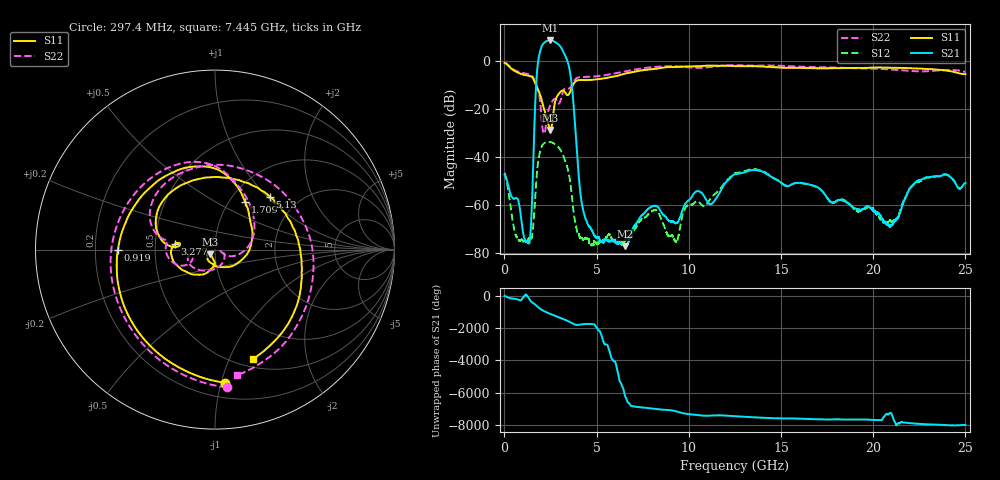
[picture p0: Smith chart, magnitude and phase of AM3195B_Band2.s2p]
!Agilent Technologies,E8364B,MY43040894,A.07.50.67
!Agilent E8364B: A.07.50.67
!Date: Wednesday, July 07, 2021 13:16:47
!Correction: S11(Full 2 Port(1,2))
!S21(Full 2 Port(1,2))
!S12(Full 2 Port(1,2))
!S22(Full 2 Port(1,2))
!S2P File: Measurements: S11, S21, S12, S22:
# Hz S  dB  R 50
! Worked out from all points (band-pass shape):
!   8001 points, 10 MHz to 25 GHz, reference 50 ohm
!   highest |S21| = 8.66 dB at 2.475 GHz (marker M1); lowest = -77.1 dB at 6.539 GHz (marker M2)
!   |S21| within 3 dB of the highest: 1.994 GHz to 3.073 GHz (1.079 GHz wide, 42.6 % of centre)
!   lowest |S11| = -28.7 dB at 2.478 GHz (marker M3), VSWR 1.08, Z = 47.4 - j2.49 ohm
!   |S11| at or under -10 dB: 1.706 GHz to 3.708 GHz (2.002 GHz wide, 73.9 % of centre)
!   |S22| runs from -30.2 to -0.5 dB; largest |S21 - S12| = 2.7
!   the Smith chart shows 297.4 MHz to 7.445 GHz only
!   S11 on the Smith chart (normalised r, x): 297.4 MHz: 0.31, -1.03; 919 MHz: 0.30, -0.00; 1.709 GHz: 1.18, +0.70; 3.277 GHz: 0.63, +0.04; 5.13 GHz: 1.44, +1.03; 7.445 GHz: 0.59, -1.23
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1e7  -0.75 -14.5  -47.39 -12.2  -46.58 -18.6  -0.51 -15.3
2.97385e8  -2.57 -85.6  -54.63 -152.2  -58.78 -157.9  -2.27 -85.2
9.190112e8  -5.33 -179.7  -66.32 99.8  -74.21 -69.9  -4.76 -179.7
1.371955e9  -6.16 121.7  -75.03 118.3  -73.86 37.3  -5.53 123.7
1.70932e9  -10.06 57.5  -11.28 123.5  -52.31 -50.5  -9.42 58.7
1.95922e9  -14.53 -3.1  4.85 -112.1  -36.96 77.6  -18.66 -16.9
2.090418e9  -18.17 -51.4  7.13 158.1  -34.70 -10.9  -29.03 -19.4
2.230986e9  -22.07 -103.9  8.15 77.2  -33.85 -90.3  -27.95 -14.8
2.474639e9  -28.66 -135.5  8.66 -42.9  -33.70 150.7  -18.55 -102.8
2.477762e9  -28.66 -134.7  8.66 -44.4  -33.70 149.3  -18.50 -103.6
2.768271e9  -16.27 -115.6  7.91 -174.7  -34.77 20.7  -15.85 -160.3
2.980686e9  -13.26 -149.6  6.62 91.0  -36.29 -71.4  -17.50 -158.4
3.277442e9  -12.89 172.3  2.64 -45.9  -41.07 155.7  -11.41 -173.7
4.177082e9  -7.86 114.8  -58.42 20.0  -73.78 130.5  -6.62 113.9
5.129826e9  -7.45 44.1  -73.47 -15.0  -75.69 -74.1  -6.15 42.6
6.538638e9  -5.20 -33.5  -77.14 -74.2  -74.86 -54.5  -4.26 -38.6
7.444525e9  -3.83 -70.7  -64.39 -75.0  -65.74 -99.2  -2.97 -80.0
8.341041e9  -3.01 -103.0  -60.91 169.4  -63.23 160.6  -2.28 -115.0
1.2505e10  -2.02 140.9  -47.13 99.3  -46.69 98.8  -1.65 127.0
1.667208e10  -2.90 20.0  -51.77 -77.5  -51.77 -79.4  -2.42 3.7
2.083604e10  -2.73 -69.0  -68.44 -133.0  -66.98 -58.1  -3.40 -81.2
2.5e10  -5.40 -124.7  -50.74 -77.3  -51.68 -76.1  -4.43 -131.8
